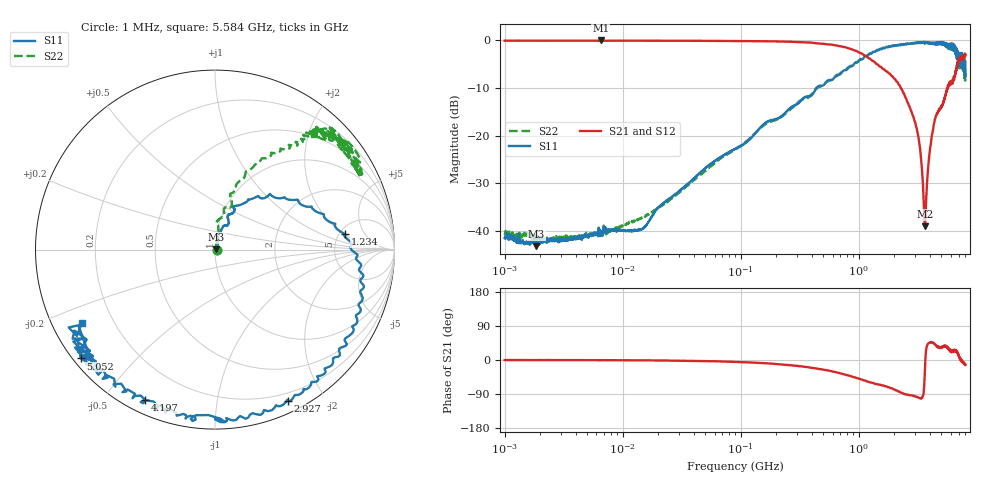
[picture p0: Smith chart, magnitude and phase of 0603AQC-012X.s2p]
!s-Parameter Generated by FASTRON Sdn. Bhd.
!FASTRON P/N : 0603AQC-012X
!Keysight Technologies: E5071C_MY46733604_B.14.02
!Date: Thu Jun 25 13:51:45 2026
!Version  :Rev00  Thu Jun 25 13:51:45 2026
!Data & Calibration Information:
!Freq  S11:SOLT2(ON)  S21:SOLT2(ON)  S12:SOLT2(ON)  S22:SOLT2(ON)
!PortZ  Port1:50+j0  Port2:50+j0
!When reading reference impedance value at option line is always used.
! Remarks : This data is being provided solely for informational purposes.
# Hz S dB R 50
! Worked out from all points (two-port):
!   1601 points, 1 MHz to 8 GHz, reference 50 ohm
!   highest |S21| = -0.03 dB at 6.532 MHz (marker M1); lowest = -39.0 dB at 3.629 GHz (marker M2)
!   |S21| within 3 dB of the highest: start of sweep to 1.095 GHz; 7.84268 GHz to 7.851731 GHz (9.051 MHz wide, 0.115 % of centre)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
!   lowest |S11| = -43.2 dB at 1.85 MHz (marker M3), VSWR 1.01, Z = 50.7 + j0.143 ohm
!   |S11| at or under -10 dB: start of sweep to 438.9 MHz
!   |S22| runs from -42.4 to -0.4 dB; largest |S21 - S12| = 0.018
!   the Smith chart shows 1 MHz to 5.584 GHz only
!   S11 on the Smith chart (normalised r, x): 1 MHz: 1.02, +0.00; 1.234 GHz: 5.58, +2.07; 2.927 GHz: 0.12, -1.58; 4.197 GHz: 0.06, -0.64; 5.052 GHz: 0.02, -0.35; 5.584 GHz: 0.09, -0.26
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1000000  -41.50 0.6  -0.08 -0.1  -0.08 -0.1  -40.80 0.3
1850129  -43.20 11.8  -0.07 -0.2  -0.08 -0.1  -41.10 4.1
4479405  -41.20 21.4  -0.08 -0.3  -0.09 -0.3  -41.20 24.2
6531720  -40.80 24.7  -0.03 -0.4  -0.13 -0.5  -40.80 32.7
1.449233e7  -39.70 44.5  -0.08 -0.9  -0.10 -0.9  -37.20 47.3
2.00676e7  -35.10 50.3  -0.09 -1.2  -0.10 -1.1  -35.20 63.4
8.994653e7  -22.80 78.5  -0.13 -4.9  -0.14 -4.9  -22.90 74.5
4.006501e8  -11.50 65.3  -0.50 -20.7  -0.50 -20.7  -11.30 69.9
8.295903e8  -5.53 31.7  -1.73 -41.4  -1.74 -41.5  -5.63 64.8
1.233539e9  -2.75 6.9  -3.82 -58.1  -3.83 -58.2  -2.93 54.8
1.7949e9  -1.33 -17.5  -6.94 -71.8  -6.97 -72.1  -1.31 50.5
2.927065e9  -0.59 -64.3  -16.40 -95.2  -16.40 -95.1  -0.61 46.2
3.26428e9  -0.41 -78.8  -21.70 -100.0  -21.70 -99.9  -0.53 43.0
3.629119e9  -0.64 -96.6  -39.00 -30.4  -38.90 -30.9  -0.50 39.2
4.196646e9  -0.70 -115.0  -19.40 46.4  -19.40 46.1  -0.74 41.2
4.716529e9  -0.66 -136.0  -14.80 33.4  -14.80 33.1  -0.88 27.3
5.052431e9  -0.32 -141.0  -14.00 33.2  -14.00 32.9  -0.63 33.0
5.584277e9  -1.42 -151.0  -10.10 35.3  -10.10 35.0  -1.42 49.5
6.110812e9  -0.99 -172.0  -8.92 20.0  -8.90 19.7  -1.57 33.7
6.766244e9  -3.76 -173.0  -5.18 22.9  -5.15 22.3  -3.79 60.0
7.383122e9  -3.69 142.0  -3.91 -3.6  -3.93 -4.4  -4.65 35.3
8e9  -4.49 138.0  -3.18 -13.0  -3.21 -13.6  -6.19 48.2
